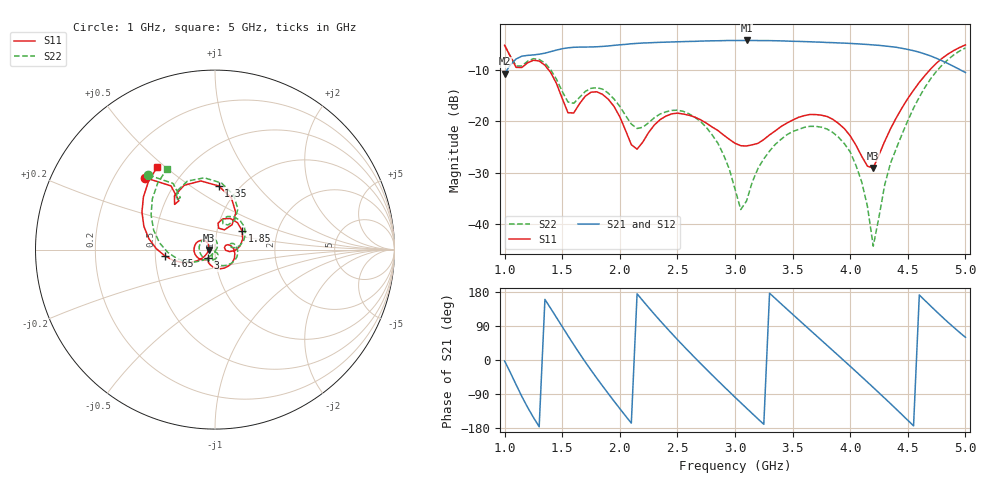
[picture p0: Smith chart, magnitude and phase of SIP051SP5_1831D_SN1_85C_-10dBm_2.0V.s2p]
# GHz  S  dB  R  50
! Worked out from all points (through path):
!   81 points, 1 GHz to 5 GHz, reference 50 ohm
!   highest |S21| = -4.14 dB at 3.1 GHz (marker M1); lowest = -10.6 dB at 1 GHz (marker M2)
!   lowest |S11| = -29.1 dB at 4.2 GHz (marker M3), VSWR 1.07, Z = 46.6 - j0.221 ohm
!   |S11| at or under -10 dB: 1.386 GHz to 4.688 GHz (3.302 GHz wide, 109 % of centre)
!   |S22| runs from -44.4 to -5.1 dB; largest |S21 - S12| = 0.0021
!   S11 on the Smith chart (normalised r, x): 1 GHz: 0.33, +0.38; 1.35 GHz: 0.80, +0.65; 1.85 GHz: 1.32, +0.29; 3 GHz: 0.92, -0.09; 4.65 GHz: 0.56, -0.04; 5 GHz: 0.35, +0.47
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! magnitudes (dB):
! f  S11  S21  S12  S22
! 1 GHz  -5.1  -10.6  -10.6  -5.1
! 1.1 GHz  -9.4  -7.8  -7.8  -9.2
! 1.35 GHz  -9.0  -6.6  -6.6  -8.6
! 1.55 GHz  -18.3  -5.6  -5.6  -16.2
! 1.7 GHz  -15.1  -5.4  -5.4  -14.1
! 1.85 GHz  -14.7  -5.3  -5.3  -13.7
! 2.15 GHz  -25.4  -4.7  -4.7  -21.4
! 2.35 GHz  -19.6  -4.5  -4.5  -18.5
! 2.7 GHz  -19.7  -4.3  -4.3  -20.0
! 2.85 GHz  -21.7  -4.2  -4.2  -24.2
! 3 GHz  -24.3  -4.2  -4.1  -33.2
! 3.05 GHz  -24.8  -4.2  -4.1  -37.2
! 3.1 GHz  -24.8  -4.1  -4.1  -35.6
! 3.2 GHz  -24.3  -4.2  -4.1  -29.2
! 3.35 GHz  -21.8  -4.2  -4.2  -24.5
! 3.7 GHz  -18.7  -4.4  -4.4  -21.0
! 4 GHz  -22.8  -4.7  -4.7  -26.0
! 4.1 GHz  -26.8  -4.9  -4.8  -31.8
! 4.2 GHz  -29.1  -5.0  -5.0  -44.4
! 4.35 GHz  -21.4  -5.3  -5.3  -28.1
! 4.65 GHz  -11.0  -6.8  -6.8  -13.3
! 5 GHz  -5.0  -10.4  -10.4  -5.6
